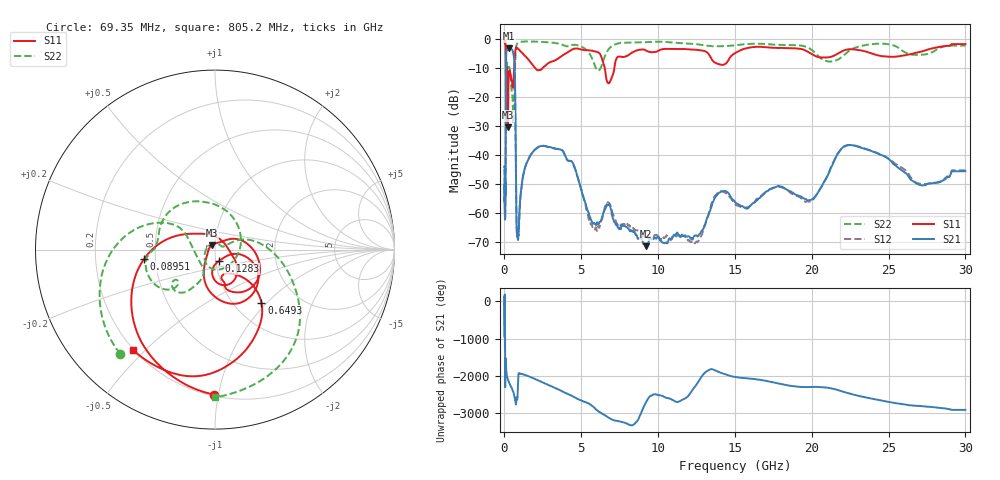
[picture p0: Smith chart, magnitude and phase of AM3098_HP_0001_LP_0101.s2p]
! Date/Time: Thu, Feb 28, 2019 8:31 AM
! Network Analyzer: Agilent Technologies E8364B Rev: A.07.50.67
! Sweep from 0.010 to 30.000 GHz, 1601 Points, Sweep Type: LOG
! Power Supply: 5.022 V, 0.002 A
# Hz S DB R 50
!freq MagS11 AngS11 MagS21 AngS21 MagS12 AngS12 MagS22 AngS22
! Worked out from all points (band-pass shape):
!   1601 points, 10 MHz to 30 GHz, reference 50 ohm
!   highest |S21| = -3.05 dB at 265.1 MHz (marker M1); lowest = -71.4 dB at 9.21 GHz (marker M2)
!   |S21| within 3 dB of the highest: 104.6 MHz to 618.5 MHz (513.9 MHz wide, 142 % of centre)
!   lowest |S11| = -30.3 dB at 227 MHz (marker M3), VSWR 1.06, Z = 48.1 + j2.35 ohm
!   |S11| at or under -10 dB: 175.9 MHz to 632 MHz (456.1 MHz wide, 113 % of centre); 2.021 GHz to 2.457 GHz (435.8 MHz wide, 19.5 % of centre); 6.531 GHz to 7.15 GHz (619.6 MHz wide, 9.06 % of centre)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
!   |S22| runs from -29.1 to -0.5 dB; largest |S21 - S12| = 0.011
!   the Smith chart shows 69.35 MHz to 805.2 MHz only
!   S11 on the Smith chart (normalised r, x): 69.35 MHz: 0.21, -0.97; 89.51 MHz: 0.43, -0.05; 128.3 MHz: 1.04, -0.13; 649.3 MHz: 1.32, -0.93; 805.2 MHz: 0.20, -0.46
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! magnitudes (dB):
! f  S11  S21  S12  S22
! 10 MHz  -0.3  -44.0  -45.6  -0.5
! 38.04 MHz  -0.5  -58.8  -60.8  -0.9
! 69.35 MHz  -1.8  -51.6  -51.7  -2.1
! 89.51 MHz  -8.0  -18.9  -18.9  -9.5
! 98.93 MHz  -24.0  -7.8  -7.8  -17.0
! 128.3 MHz  -23.5  -4.0  -4.0  -11.1
! 144.7 MHz  -13.3  -3.6  -3.6  -10.1
! 185.8 MHz  -11.3  -3.5  -3.5  -8.1
! 227 MHz  -30.3  -3.1  -3.1  -9.5
! 265.1 MHz  -14.6  -3.1  -3.0  -9.8
! 550.5 MHz  -16.7  -4.1  -4.1  -24.7
! 649.3 MHz  -8.1  -8.4  -8.4  -18.4
! 805.2 MHz  -2.8  -65.9  -66.8  -1.7
! 2.084 GHz  -10.4  -37.6  -37.6  -0.7
! 3.76 GHz  -5.6  -38.4  -38.2  -1.7
! 5.783 GHz  -3.9  -63.5  -64.6  -7.6
! 6.821 GHz  -15.0  -56.9  -56.8  -3.1
! 7.926 GHz  -5.8  -64.8  -63.3  -1.1
! 9.21 GHz  -3.8  -71.4  -67.9  -0.9
! 19.8 GHz  -4.4  -55.5  -56.1  -2.9
! 22.56 GHz  -3.4  -36.5  -36.5  -3.5
! 30 GHz  -1.6  -45.5  -45.2  -2.1
